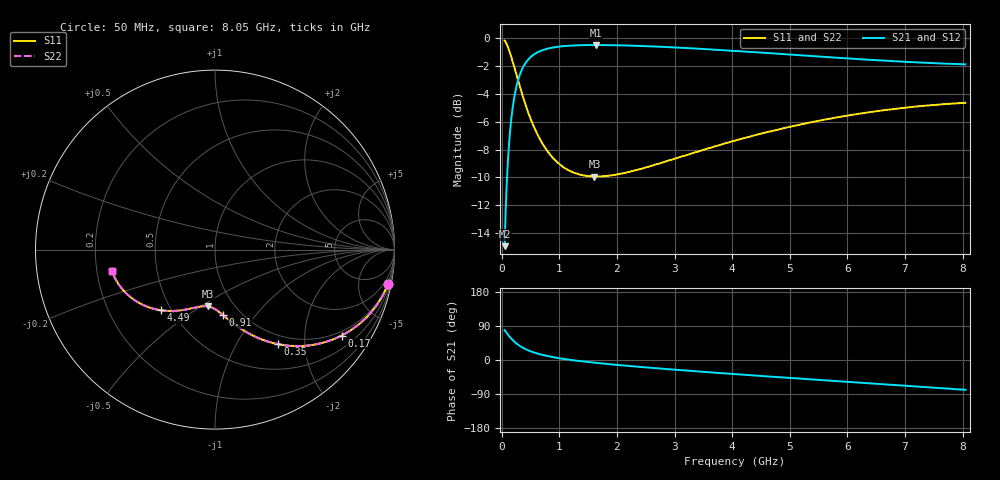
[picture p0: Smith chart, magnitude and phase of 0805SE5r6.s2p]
! AVX Thin Film Operation		Date: August 2001
! Description: Accu-P® Series, Thin Film, SMD, RF Capacitor
! Part Number: 08051J5R6ABT
! 50 MHz  -  8.05 GHz
! Serial Measurements
# mhz S db R 50
!	S11		S21		S12		S22
!	dB	Phase	dB	Phase	dB	Phase	dB	Phase
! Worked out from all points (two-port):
!   401 points, 50 MHz to 8.05 GHz, reference 50 ohm
!   highest |S21| = -0.47 dB at 1.63 GHz (marker M1); lowest = -14.9 dB at 50 MHz (marker M2)
!   |S21| within 3 dB of the highest: 254.8 MHz to end of sweep
!   lowest |S11| = -9.9 dB at 1.61 GHz (marker M3), VSWR 1.94, Z = 38.1 - j26.8 ohm
!   |S11| at or under -10 dB: nowhere
!   |S22| runs from -9.9 to -0.1 dB; largest |S21 - S12| = 0
!   S11 on the Smith chart (normalised r, x): 50 MHz: 1, -10; 170 MHz: 0.86, -3.03; 350 MHz: 0.86, -1.51; 910 MHz: 0.83, -0.70; 4.49 GHz: 0.44, -0.37; 8.05 GHz: 0.26, -0.09
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50  -0.14 -11.1  -14.95 78.9  -14.95 78.9  -0.14 -11.1
90  -0.44 -19.5  -10.16 70.5  -10.16 70.5  -0.44 -19.5
130  -0.87 -27.3  -7.42 62.7  -7.42 62.7  -0.87 -27.3
170  -1.38 -34.2  -5.64 55.8  -5.64 55.8  -1.38 -34.2
210  -1.95 -40.3  -4.42 49.7  -4.42 49.7  -1.95 -40.3
250  -2.53 -45.7  -3.55 44.3  -3.55 44.3  -2.53 -45.7
350  -3.95 -56.2  -2.24 33.8  -2.24 33.8  -3.95 -56.2
450  -5.21 -63.9  -1.56 26.1  -1.56 26.1  -5.21 -63.9
570  -6.46 -70.7  -1.12 19.2  -1.12 19.2  -6.46 -70.7
710  -7.58 -76.6  -0.84 13.3  -0.84 13.3  -7.58 -76.7
910  -8.69 -83.0  -0.64 7.0  -0.64 7.0  -8.69 -83.0
1130  -9.42 -88.3  -0.53 1.7  -0.53 1.7  -9.42 -88.3
1390  -9.83 -93.3  -0.48 -3.4  -0.48 -3.4  -9.83 -93.3
1610  -9.93 -97.0  -0.47 -7.1  -0.47 -7.1  -9.93 -97.1
1630  -9.93 -97.4  -0.47 -7.4  -0.47 -7.4  -9.93 -97.4
2150  -9.66 -104.9  -0.50 -15.0  -0.50 -15.0  -9.66 -104.9
2730  -9.00 -112.2  -0.59 -22.3  -0.59 -22.3  -9.00 -112.2
4050  -7.35 -127.2  -0.89 -37.3  -0.89 -37.3  -7.35 -127.2
4490  -6.86 -131.9  -1.01 -42.0  -1.01 -42.0  -6.86 -131.9
5390  -6.01 -141.2  -1.26 -51.4  -1.26 -51.4  -6.01 -141.3
6730  -5.11 -154.9  -1.62 -65.0  -1.62 -65.0  -5.11 -154.9
8050  -4.63 -168.5  -1.86 -78.7  -1.86 -78.7  -4.63 -168.5
